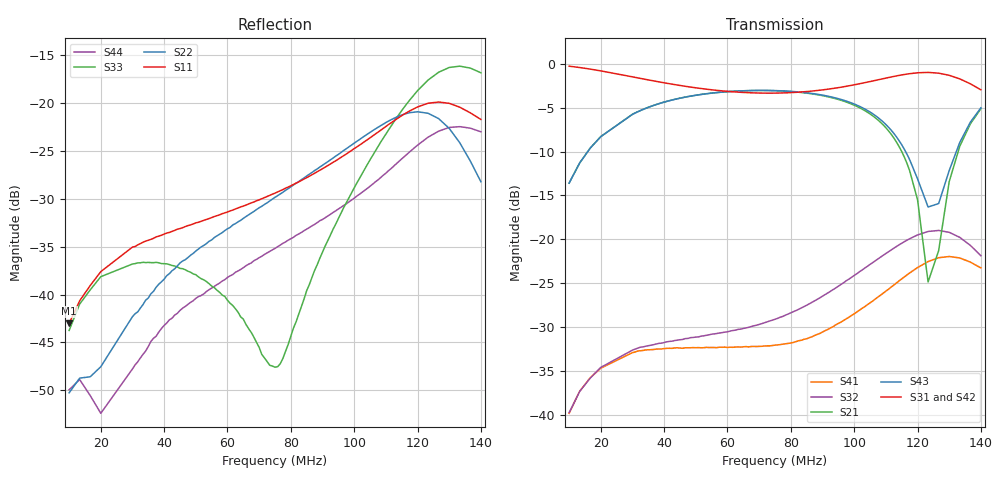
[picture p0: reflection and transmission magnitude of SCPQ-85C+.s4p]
!Agilent Technologies,N5230A,US43500299,A.07.50.26
!Agilent N5230A: A.07.50.26
!Date: Thursday, May 31, 2012 15:50:31
!Correction: S11(Full 4 Port(1,2,3,4))
!S12(Full 4 Port(1,2,3,4))
!S13(Full 4 Port(1,2,3,4))
!S14(Full 4 Port(1,2,3,4))
!S21(Full 4 Port(1,2,3,4))
!S22(Full 4 Port(1,2,3,4))
!S23(Full 4 Port(1,2,3,4))
!S24(Full 4 Port(1,2,3,4))
!S31(Full 4 Port(1,2,3,4))
!S32(Full 4 Port(1,2,3,4))
!S33(Full 4 Port(1,2,3,4))
!S34(Full 4 Port(1,2,3,4))
!S41(Full 4 Port(1,2,3,4))
!S42(Full 4 Port(1,2,3,4))
!S43(Full 4 Port(1,2,3,4))
!S44(Full 4 Port(1,2,3,4))
!S4P File: Measurements: <S11,S12,S13,S14>,
!Port1-Sum; Port2-+90 degree port; Port3-0 degree port; Port4-Term
!<S21,S22,S23,S24>,
!<S31,S32,S33,S34>,
!<S41,S42,S43,S44>:
# Hz S  dB  R 50
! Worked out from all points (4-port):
!   117 points, 10 MHz to 140 MHz, reference 50 ohm
!   strongest paths, dB at 10 MHz, 50.83 MHz, 75 MHz, 99.17 MHz, 140 MHz:
!     S31: -0.2, -2.8, -3.3, -2.4, -2.9
!     S42: -0.3, -2.8, -3.3, -2.4, -2.9
!     S43: -13.6, -3.5, -3.0, -4.4, -5.0
!     S21: -13.6, -3.5, -3.0, -4.6, -5.1
!     S32: -39.8, -31.1, -29.1, -24.3, -21.9
!     S41: -39.9, -32.4, -32.1, -28.7, -23.3
!   lowest |S11| = -43.0 dB at 10 MHz (marker M1), VSWR 1.01, Z = 49.9 - j0.701 ohm
!   |S11| at or under -10 dB: start of sweep to end of sweep
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1e7  -43.01 -97.0  -13.59 74.5  -0.25 -15.2  -39.84 69.5
     -13.59 74.5  -50.26 -49.8  -39.75 69.9  -0.25 -15.5
     -0.25 -15.2  -39.79 70.1  -43.75 -98.9  -13.59 74.7
     -39.86 69.3  -0.26 -15.5  -13.59 74.7  -49.95 -37.8
4.083333e7  -33.56 172.0  -4.26 37.9  -2.20 -51.3  -32.44 19.0
            -4.26 37.9  -38.01 118.3  -31.70 18.0  -2.19 -52.5
            -2.20 -51.3  -31.70 18.1  -36.78 -162.3  -4.26 38.6
            -32.45 19.0  -2.20 -52.5  -4.27 38.6  -42.96 105.7
7.583333e7  -29.26 117.0  -3.06 10.8  -3.32 -77.8  -32.06 8.4
            -3.06 10.9  -29.65 52.1  -29.01 -4.3  -3.31 -80.1
            -3.32 -77.8  -29.02 -4.3  -47.53 -118.2  -3.03 13.0
            -32.05 8.4  -3.32 -80.2  -3.04 13.0  -34.99 31.0
1.108333e8  -22.22 63.0  -7.63 -24.4  -1.55 -114.4  -25.71 3.8
            -7.63 -24.3  -21.86 -26.3  -21.42 -57.0  -1.53 -118.0
            -1.54 -114.4  -21.43 -57.0  -22.79 -95.8  -7.20 -13.9
            -25.70 3.8  -1.54 -118.0  -7.21 -13.9  -27.05 -26.2
1.2e8  -20.38 38.1  -15.50 -35.8  -1.01 -132.4  -23.24 -13.1
       -15.49 -35.8  -20.89 -64.8  -19.50 -92.3  -0.96 -136.3
       -1.00 -132.4  -19.51 -92.3  -18.68 -123.9  -13.10 -9.6
       -23.23 -13.1  -0.97 -136.3  -13.10 -9.6  -24.38 -48.9
1.233333e8  -19.99 27.5  -24.87 -20.6  -0.96 -140.2  -22.56 -22.3
            -24.87 -20.6  -21.04 -82.0  -19.11 -108.2  -0.91 -144.2
            -0.96 -140.2  -19.11 -108.2  -17.57 -136.8  -16.32 12.3
            -22.55 -22.2  -0.92 -144.2  -16.32 12.3  -23.54 -59.7
1.4e8  -21.69 -20.3  -5.11 81.8  -2.95 178.8  -23.29 -71.9
       -5.10 81.8  -28.20 162.8  -21.87 161.3  -2.86 173.7
       -2.95 178.8  -21.88 161.3  -16.81 154.0  -5.00 69.8
       -23.27 -71.9  -2.86 173.7  -5.00 69.8  -22.98 -124.1
